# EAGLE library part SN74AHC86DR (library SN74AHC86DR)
Quadruple 2-Input Exclusive-OR Gates Source: Datasheet
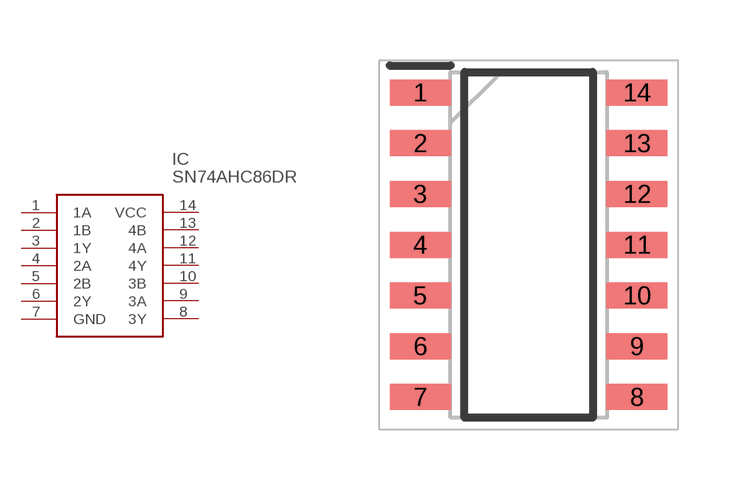
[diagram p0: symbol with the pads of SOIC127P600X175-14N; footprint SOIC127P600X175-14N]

Designator prefix IC

## SN74AHC86DR (Description: Quadruple 2-Input Exclusive-OR Gates; Height: 1.75mm; Manufacturer_Name: Texas Instruments; Manufacturer_Part_Number: SN74AHC86DR; Mouser_Part_Number: 595-SN74AHC86DR; Mouser_Price-Stock: https://www.mouser.co.uk/ProductDetail/Texas-Instruments/SN74AHC86DR?qs=D5pVkbrsqqK0yvWJ8LFETg%3D%3D)  [SOIC127P600X175-14N]
1  1A
2  1B
3  1Y
4  2A
5  2B
6  2Y
7  GND
8  3Y
9  3A
10  3B
11  4Y
12  4A
13  4B
14  VCC

## Footprint SOIC127P600X175-14N (pad centres in mm)
D (-R-PDSO-G14)
smd 1.525 x 0.65: 1 -2.712,3.81; 2 -2.712,2.54; 3 -2.712,1.27; 4 -2.712,0; 5 -2.712,-1.27; 6 -2.712,-2.54; 7 -2.712,-3.81; 8 2.712,-3.81; 9 2.712,-2.54; 10 2.712,-1.27; 11 2.712,0; 12 2.712,1.27; 13 2.712,2.54; 14 2.712,3.81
